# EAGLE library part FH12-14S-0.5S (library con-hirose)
0.5mm Pitch Connectors For FPC/FFC Source: Data sheet
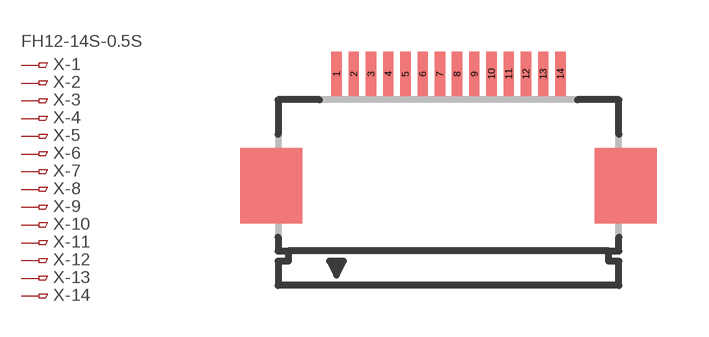
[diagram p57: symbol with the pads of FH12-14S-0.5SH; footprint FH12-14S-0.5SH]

Designator prefix X; gates -1=PINV -2=PIN -3=PIN -4=PIN -5=PIN -6=PIN -7=PIN -8=PIN -9=PIN -10=PIN -11=PIN -12=PIN -13=PIN -14=PIN

## FH12-14S-0.5SH (MPN: MC34827; OC_FARNELL: 1324544; OC_NEWARK: 41P0493)  [FH12-14S-0.5SH]
1  -1:1  pas
2  -2:1  pas
3  -3:1  pas
4  -4:1  pas
5  -5:1  pas
6  -6:1  pas
7  -7:1  pas
8  -8:1  pas
9  -9:1  pas
10  -10:1  pas
11  -11:1  pas
12  -12:1  pas
13  -13:1  pas
14  -14:1  pas

## Footprint FH12-14S-0.5SH (pad centres in mm)
0.5mm Pitch Connectors For FPC/FFC Source: Data sheet
smd 0.3 x 1.3: 1 -3.25,3.25; 2 -2.75,3.25; 3 -2.25,3.25; 4 -1.75,3.25; 5 -1.25,3.25; 6 -0.75,3.25; 7 -0.25,3.25; 8 0.25,3.25; 9 0.75,3.25; 10 1.25,3.25; 11 1.75,3.25; 12 2.25,3.25; 13 2.75,3.25; 14 3.25,3.25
